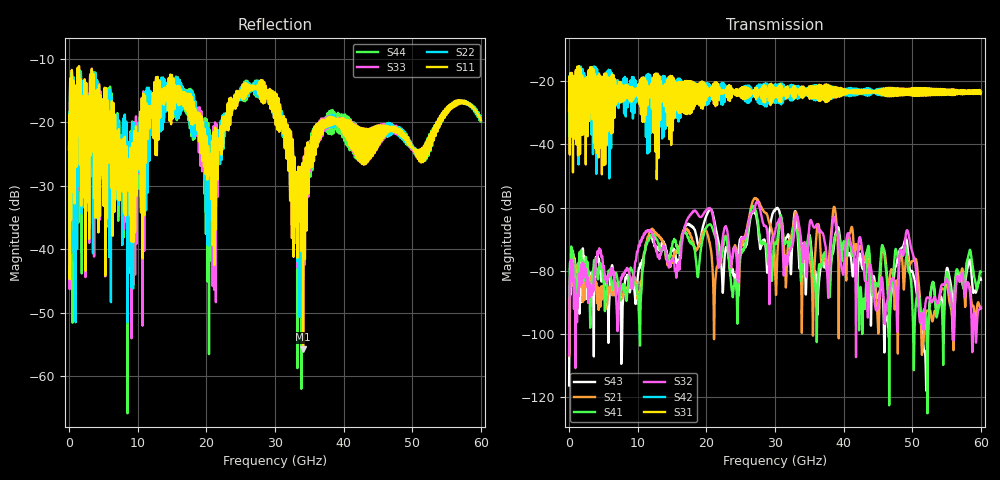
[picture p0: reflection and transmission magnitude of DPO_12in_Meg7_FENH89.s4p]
! Touchstone data
! Created: 10-Dec-2018 by IdEM R2012 (8.0.5)
# Hz S MA R 50
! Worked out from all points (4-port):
!   6000 points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, 10 MHz to 60 GHz, reference 50 ohm
!   strongest paths, dB at 10 MHz, 15.01 GHz, 30.01 GHz, 45.01 GHz, 60 GHz:
!     S31: -29.5, -18.5, -22.3, -23.1, -23.9
!     S42: -29.5, -23.8, -21.3, -22.6, -23.2
!     S32: -106.7, -76.5, -67.9, -91.5, -91.5
!     S41: -102.0, -72.4, -71.4, -85.0, -80.4
!     S21: -106.9, -77.4, -80.1, -98.3, -91.9
!     S43: -116.3, -73.5, -60.9, -87.9, -82.9
!   lowest |S11| = -55.8 dB at 34.1 GHz (marker M1), VSWR 1.00, Z = 50.1 + j0.0985 ohm
!   |S11| at or under -10 dB: start of sweep to end of sweep
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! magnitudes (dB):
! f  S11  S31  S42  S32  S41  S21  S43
! 10 MHz  -24.2  -29.5  -29.5  -106.7  -102.0  -106.9  -116.3
! 20.36 GHz  -27.3  -22.8  -21.6  -60.2  -65.5  -70.4  -60.9
! 24.73 GHz  -16.2  -23.2  -22.8  -79.0  -80.8  -87.8  -72.7
! 27.17 GHz  -14.4  -22.5  -22.5  -59.1  -60.9  -57.2  -62.2
! 34.1 GHz  -55.8  -22.8  -22.7  -76.5  -74.3  -77.3  -71.3
! 38.63 GHz  -19.4  -24.9  -22.1  -62.9  -70.1  -59.8  -71.6
! 60 GHz  -19.7  -23.9  -23.2  -91.5  -80.4  -91.9  -82.9
